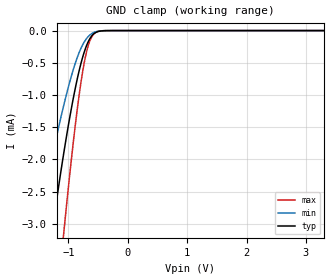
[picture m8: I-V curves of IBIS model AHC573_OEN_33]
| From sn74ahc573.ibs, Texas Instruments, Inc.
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[Model]   AHC573_OEN_33
Model_type  Input
Vinl=0.9
Vinh=2.1
| variable   typ   min   max
C_comp   0.76pF   0.68pF   0.83pF
[Temperature Range]   40   100   -40
| Ambient temperature   25   85   -40
[Voltage range]   3.3   3   3.6
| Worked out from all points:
|   GND clamp passes 1 mA (typ) near -0.91 V on its own axis
[GND Clamp]
| AHC573_OEN_33
|   Voltage   I(typ)   I(min)   I(max)
-3.3V     -21.16mA   -13.87mA   -28.72mA
-1.52V    -4.862mA   -3.111mA   -7.657mA
-1.28V    -3.16mA    -1.99mA    -5.12mA
-1.245V   -2.93mA    -1.837mA   -4.764mA
-1.1V     -2.029mA   -1.242mA   -3.345mA
-1.07V    -1.855mA   -1.127mA   -3.064mA
-905mV    -991.3uA   -567.1uA   -1.632mA
-780mV    -480.2uA   -258.6uA   -751.8uA
-690mV    -222.9uA   -118.9uA   -313.8uA
-590mV    -64.59uA   -38.15uA   -73.91uA
-375mV    -1.358uA   -994.5nA   -683.1nA
3.3V      3.761nA    612.9pA    18.13nA
